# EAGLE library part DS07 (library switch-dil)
DIL/CODE SWITCH
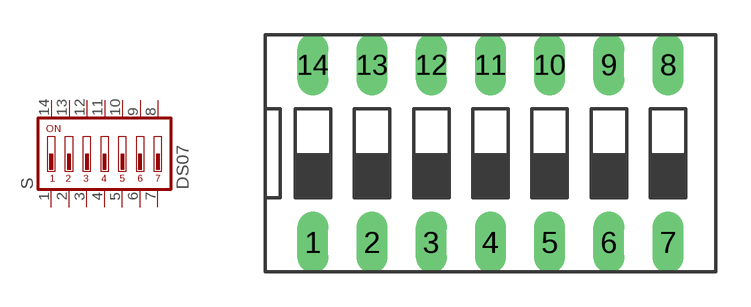
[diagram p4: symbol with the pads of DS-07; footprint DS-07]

Designator prefix S

## DS07 (MPN: MCDS07; OC_FARNELL: 1255226; OC_NEWARK: 26M1106)  [DS-07]
1  1  pas
2  2  pas
3  3  pas
4  4  pas
5  5  pas
6  6  pas
7  7  pas
8  8  pas
9  9  pas
10  10  pas
11  11  pas
12  12  pas
13  13  pas
14  14  pas

## Footprint DS-07 (pad centres in mm)
DIL/CODE SWITCH Mors distributor Buerklin, 17G560
drill 0.813 long: 1 -7.62,-3.81; 2 -5.08,-3.81; 3 -2.54,-3.81; 4 0,-3.81; 5 2.54,-3.81; 6 5.08,-3.81; 7 7.62,-3.81; 8 7.62,3.81; 9 5.08,3.81; 10 2.54,3.81; 11 0,3.81; 12 -2.54,3.81; 13 -5.08,3.81; 14 -7.62,3.81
